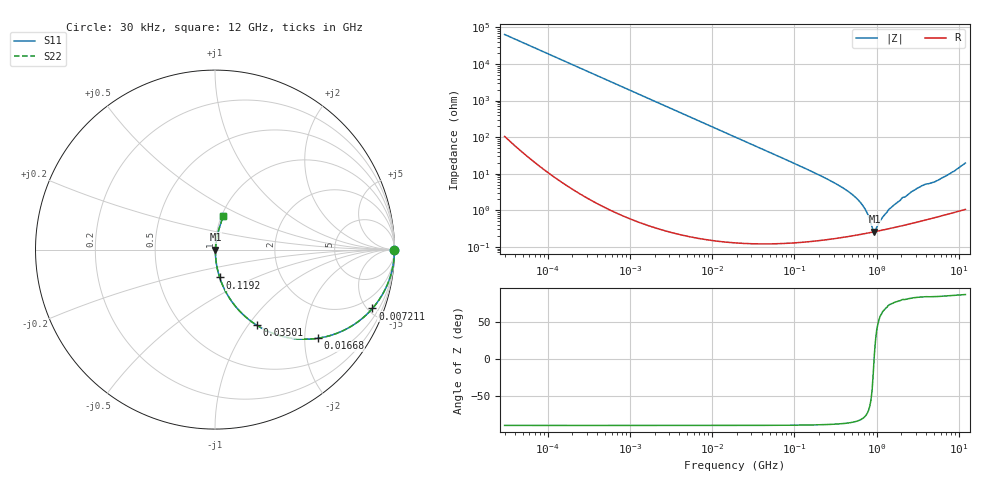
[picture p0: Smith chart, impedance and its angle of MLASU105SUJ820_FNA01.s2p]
! MLASU105SUJ820_FNA01  S-PARAMETER MODEL  ( General Type )
! Model Generated by TAIYO YUDEN Corporation (http://www.ty-top.com)
! Version 4.0
! TAIYO YUDEN Control No. 120810
! Copyright(c) 2003 TAIYO YUDEN CO.,LTD. All Rights Reserved.
! Product Description (link to TY-COMPAS)
! https://ds.yuden.co.jp/TYCOMPAS/or/detail?pn=MLASU105SUJ820JFNA01&u=M
! Products Name : Multilayer Ceramic Capacitors
! Characteristics :
!  Capacitance : 82 pF , Rated Voltage : 50V , TCC : UJ / U2J
!  Case Size : 1.0 x 0.5 / 0.039 x 0.02 [mm/inch] , Thickness : 0.5 / 0.02 [mm/inch]
!  (Conditions: Temperature = 25 degC , DC Bias Current/Voltage = 0A / 0V)
! External Node Assignments :
!  1  o---| |---o  2
! GND o---------o GND
! Frequency Range : 0.03MHz  -  12000MHz  [ 401 STEP ]
# MHz S RI R 50
! Freq[MHz].  S11 Real  S11 Imag  S21 Real  S21 Imag  S12 Real  S12 Imag  S22 Real  S22 Imag
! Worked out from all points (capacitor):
!   401 points, 30 kHz to 12 GHz, reference 50 ohm
!   read as one part in series: C = 82.4 pF near 32 kHz
!   lowest |Z| = 260 mohm at 939.2 MHz (marker M1)
!   series resonance near 932.3 MHz, so ESL is about 350 pH
!   S11 on the Smith chart (normalised r, x): 30 kHz: open; 7.211 MHz: 1.00, -5.36; 16.68 MHz: 1.00, -2.32; 35.01 MHz: 1.00, -1.10; 119.2 MHz: 1.00, -0.32; 12 GHz: 1.02, +0.39
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0.03  1 -0.00155  4.95e-06 0.00155  4.95e-06 0.00155  1 -0.00155
0.260295  0.9998 -0.0135  0.000186 0.0135  0.000186 0.0135  0.9998 -0.0135
2.258455  0.9865 -0.1154  0.0135 0.1154  0.0135 0.1154  0.9865 -0.1154
7.211021  0.8775 -0.3276  0.1225 0.3276  0.1225 0.3276  0.8775 -0.3276
10.96639  0.7559 -0.4291  0.2441 0.4291  0.2441 0.4291  0.7559 -0.4291
16.67749  0.5726 -0.4941  0.4274 0.4941  0.4274 0.4941  0.5726 -0.4941
18.97367  0.5086 -0.4993  0.4914 0.4993  0.4914 0.4993  0.5086 -0.4993
35.01459  0.2332 -0.4218  0.7668 0.4218  0.7668 0.4218  0.2332 -0.4218
60.58103  0.0924 -0.2877  0.9076 0.2877  0.9076 0.2877  0.0924 -0.2877
119.2463  0.026 -0.1549  0.974 0.1549  0.974 0.1549  0.026 -0.1549
164.6252  0.0141 -0.1119  0.9859 0.1119  0.9859 0.1119  0.0141 -0.1119
356.9603  0.00387 -0.0459  0.9961 0.0459  0.9961 0.0459  0.00387 -0.0459
560.6502  0.00255 -0.0219  0.9974 0.0219  0.9974 0.0219  0.00255 -0.0219
725.66  0.00241 -0.0104  0.9976 0.0104  0.9976 0.0104  0.00241 -0.0104
799.3715  0.00244 -0.00632  0.9976 0.00632  0.9976 0.00632  0.00244 -0.00632
880.5704  0.00251 -0.0023  0.9975 0.0023  0.9975 0.0023  0.00251 -0.0023
939.2353  0.00258 0.000278  0.9974 -0.000278  0.9974 -0.000278  0.00258 0.000278
1428.372  0.00325 0.0103  0.9968 -0.0103  0.9968 -0.0103  0.00325 0.0103
2903.719  0.00579 0.0352  0.9942 -0.0352  0.9942 -0.0352  0.00579 0.0352
3758.338  0.00758 0.0482  0.9924 -0.0482  0.9924 -0.0482  0.00758 0.0482
5534.236  0.0107 0.0644  0.9893 -0.0644  0.9893 -0.0644  0.0107 0.0644
12000  0.0464 0.1851  0.9536 -0.1851  0.9536 -0.1851  0.0464 0.1851
